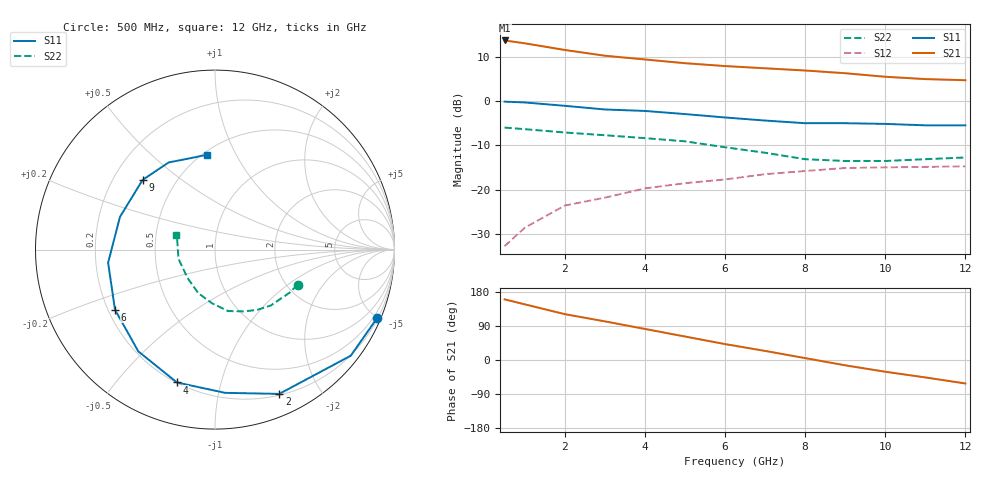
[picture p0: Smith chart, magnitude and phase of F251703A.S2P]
!ATF-25170
!S-PARAMETERS at Vds=3V  Id=20mA.  LAST UPDATED 07-22-92
# ghz s ma r 50
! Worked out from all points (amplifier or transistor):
!   13 points, 500 MHz to 12 GHz, reference 50 ohm
!   highest |S21| = 13.6 dB at 500 MHz (marker M1)
!   |S21| within 3 dB of that: start of sweep to 2.66 GHz
!   unconditionally stable (mu >= 1): 9.301 GHz to end of sweep
!   at 2 GHz: K = 0.41, MSG = 17.5 dB, |S12| = -23.6 dB
!   at 6 GHz: K = 0.91, MSG = 12.8 dB, |S12| = -17.7 dB
!   at 12 GHz: K = 1.12, MAG = 7.6 dB, |S12| = -14.8 dB
!   lowest NFmin = 0.60 dB at 500 MHz
!   S11 on the Smith chart (normalised r, x): 500 MHz: 0.25, -4.90; 2 GHz: 0.21, -1.52; 4 GHz: 0.20, -0.73; 6 GHz: 0.23, -0.26; 9 GHz: 0.32, +0.37; 12 GHz: 0.52, +0.77
0.5  0.98 -23.0  4.8 160.0  0.023 76.0  0.5 -23.0
1  0.96 -38.0  4.46 147.0  0.037 67.0  0.48 -30.0
2  0.88 -66.0  3.75 121.0  0.066 50.0  0.44 -45.0
3  0.8 -86.0  3.23 102.0  0.081 41.0  0.41 -55.0
4  0.77 -106.0  2.93 82.0  0.103 28.0  0.38 -65.0
5  0.71 -127.0  2.66 62.0  0.118 17.0  0.35 -78.0
6  0.65 -149.0  2.47 42.0  0.13 6.0  0.3 -93.0
7  0.6 -173.0  2.33 24.0  0.149 -4.0  0.26 -111.0
8  0.56 161.0  2.2 5.0  0.162 -16.0  0.22 -134.0
9  0.56 136.0  2.05 -14.0  0.175 -26.0  0.21 -166.0
10  0.55 118.0  1.87 -31.0  0.178 -35.0  0.21 173.0
11  0.53 108.0  1.76 -46.0  0.18 -42.0  0.22 164.0
12  0.53 95.0  1.71 -62.0  0.183 -52.0  0.23 159.0
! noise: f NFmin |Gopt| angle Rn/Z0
0.5  0.6  0.94  11  0.9
1  0.6  0.89  24  0.78
2  0.7  0.77  50  0.53
4  0.8  0.63  105  0.33
6  1  0.66  147  0.06
8  1.2  0.62  -159  0.11
12  1.6  0.59  -93  0.69
